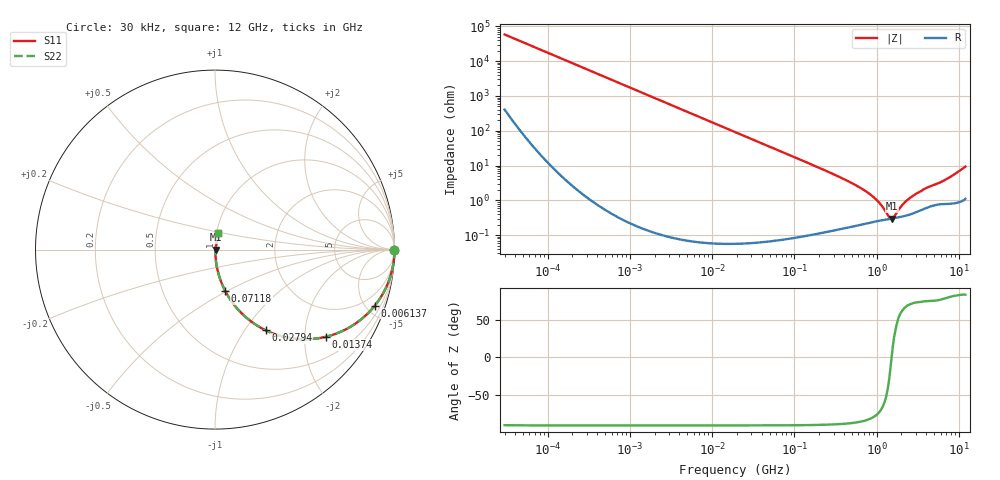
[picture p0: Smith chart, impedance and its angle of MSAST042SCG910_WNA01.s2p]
! MSAST042SCG910_WNA01  S-PARAMETER MODEL  ( General Type )
! Model Generated by TAIYO YUDEN Corporation (http://www.ty-top.com)
! Version 1.0
! TAIYO YUDEN Control No. 150820
! Copyright(c) 2015 TAIYO YUDEN CO.,LTD. All Rights Reserved.
! Product Description (link to TY-COMPAS)
! https://ds.yuden.co.jp/TYCOMPAS/or/detail?pn=MSAST042SCG910JWNA01&u=M
! Products Name : Multilayer Ceramic Capacitors
! Characteristics :
!  Capacitance : 91 pF , Rated Voltage : 25V , TCC : CG / C0G
!  Case Size : 0.4 x 0.2 / 0.016 x 0.008 [mm/inch] , Thickness : 0.2 / 0.008 [mm/inch]
!  (Conditions: Temperature = 25 degC , DC Bias Current/Voltage = 0A / 0V)
! External Node Assignments :
!  1  o---| |---o  2
! GND o---------o GND
! Frequency Range : 0.03MHz  -  12000MHz  [ 401 STEP ]
# MHz S RI R 50
! Freq[MHz].  S11 Real  S11 Imag  S21 Real  S21 Imag  S12 Real  S12 Imag  S22 Real  S22 Imag
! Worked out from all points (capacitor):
!   401 points, 30 kHz to 12 GHz, reference 50 ohm
!   read as one part in series: C = 91 pF near 32 kHz
!   lowest |Z| = 298 mohm at 1.524 GHz (marker M1)
!   series resonance near 1.522 GHz, so ESL is about 120 pH
!   S11 on the Smith chart (normalised r, x): 30 kHz: open; 6.137 MHz: 1.00, -5.70; 13.74 MHz: 1.00, -2.55; 27.94 MHz: 1.00, -1.25; 71.18 MHz: 1.00, -0.49; 12 GHz: 1.02, +0.19
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0.03  1 -0.00172  1.48e-05 0.00172  1.48e-05 0.00172  1 -0.00172
0.260295  0.9998 -0.0149  0.000225 0.0149  0.000225 0.0149  0.9998 -0.0149
2.258455  0.9836 -0.127  0.0164 0.127  0.0164 0.127  0.9836 -0.127
6.13721  0.8903 -0.3124  0.1097 0.3124  0.1097 0.3124  0.8903 -0.3124
9.037177  0.7892 -0.4077  0.2108 0.4077  0.2108 0.4077  0.7892 -0.4077
13.74358  0.6182 -0.4856  0.3818 0.4856  0.3818 0.4856  0.6182 -0.4856
18.97367  0.4593 -0.498  0.5407 0.498  0.5407 0.498  0.4593 -0.498
27.93914  0.2816 -0.4493  0.7184 0.4493  0.7184 0.4493  0.2816 -0.4493
43.88187  0.1373 -0.3434  0.8627 0.3434  0.8627 0.3434  0.1373 -0.3434
71.18072  0.0573 -0.231  0.9427 0.231  0.9427 0.231  0.0573 -0.231
164.6252  0.0119 -0.1036  0.9881 0.1036  0.9881 0.1036  0.0119 -0.1036
433.1624  0.00299 -0.0369  0.997 0.0369  0.997 0.0369  0.00299 -0.0369
749.4426  0.00247 -0.0176  0.9975 0.0176  0.9975 0.0176  0.00247 -0.0176
1068.55  0.00264 -0.00827  0.9974 0.00827  0.9974 0.00827  0.00264 -0.00827
1428.372  0.00289 -0.00147  0.9971 0.00147  0.9971 0.00147  0.00289 -0.00147
1523.532  0.00297 2.58e-05  0.997 -2.58e-05  0.997 -2.58e-05  0.00297 2.58e-05
1625.032  0.00305 0.00147  0.9969 -0.00147  0.9969 -0.00147  0.00305 0.00147
2172.242  0.00357 0.00768  0.9964 -0.00768  0.9964 -0.00768  0.00357 0.00768
2722.352  0.00427 0.0124  0.9957 -0.0124  0.9957 -0.0124  0.00427 0.0124
3881.513  0.00623 0.0207  0.9938 -0.0207  0.9938 -0.0207  0.00623 0.0207
6715.658  0.00911 0.0365  0.9909 -0.0365  0.9909 -0.0365  0.00911 0.0365
12000  0.0192 0.0898  0.9808 -0.0898  0.9808 -0.0898  0.0192 0.0898
